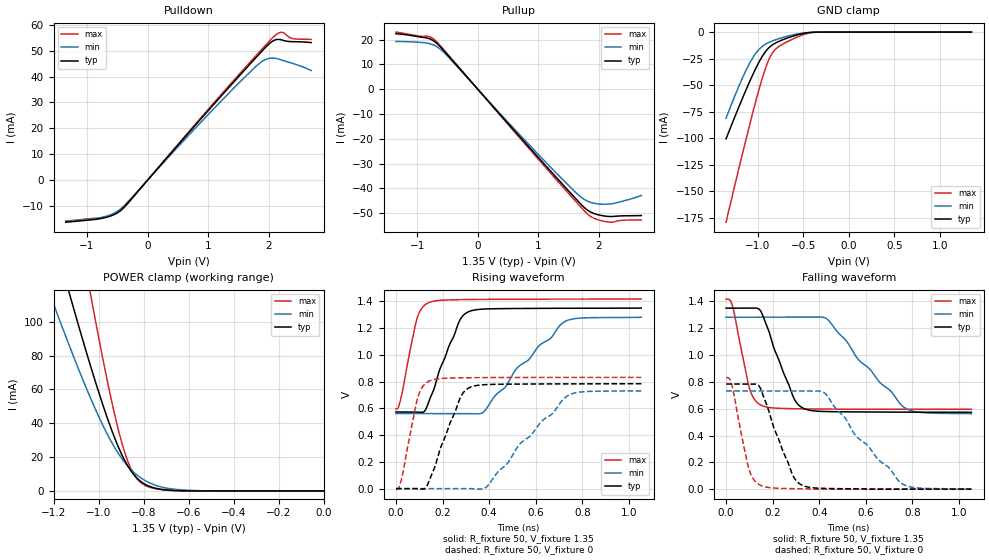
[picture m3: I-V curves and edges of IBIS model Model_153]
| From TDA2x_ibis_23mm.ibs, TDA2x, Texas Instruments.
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| Model based on original model for DDR_SEIOPB_H
|   Sub model SR010_DRV34_1P35
[model]   Model_153
|[Description]  [1.35V-I/O-X-X]
|   , ,
|[Input Load]
|[Output Drive]
|Voltage   1.35V
|Mode   I/O
Model_type   I/O
Polarity   Non-Inverting
Enable   Active-Low
Vinl =  0.585
Vinh =  0.765
Cref =  15.0000pF
Rref =  100.0000M
Vref =  0V
Vmeas =  0.675
C_comp   2p   2p   2p
[Model Spec]
Vinl   0.585   0.55125   0.61875
Vinh   0.765   0.73125   0.79875
[Receiver Thresholds]
Tslew_ac = 5n
Vth= 0.675
Vth_max= 0.709
Vth_min= 0.608
Vinh_ac= 0.175
Vinh_dc= 0.1
Vinl_ac= -0.175
Vinl_dc= -0.1
[Temperature Range]   25   125   -40
[Voltage Range]   1.35   1.2825   1.4175
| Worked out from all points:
|   slope of the pulldown table from 0 to 0.203 V, typ, clamps not added: 36.8 ohm
|   slope of the pullup table from 0 to 0.203 V, typ, clamps not added: 36 ohm
|   GND clamp passes 1 mA (typ) near -0.48 V on its own axis
|   POWER clamp passes 1 mA (typ) near -0.72 V on its own axis
|   rising waveform, R_fixture 50, V_fixture 1.35: 20-80 % time 99.6ps typ, 239ps min, 55.7ps max; typ from 0.573 V to 1.35 V
|   rising waveform, R_fixture 50, V_fixture 0: 20-80 % time 98.8ps typ, 233ps min, 55.9ps max; typ from 0 V to 0.784 V
|   falling waveform, R_fixture 50, V_fixture 1.35: 20-80 % time 99ps typ, 221ps min, 57.3ps max; typ from 1.35 V to 0.573 V
|   falling waveform, R_fixture 50, V_fixture 0: 20-80 % time 99.4ps typ, 226ps min, 56.8ps max; typ from 0.784 V to 0 V
[POWER_clamp]
-1.35V    224.4mA    165.8mA    358.5mA
-1.214V   157mA      115.5mA    250.8mA
-1.132V   117.8mA    86.59mA    187.7mA
-1.118V   111.4mA    81.92mA    177.3mA
-1.036V   74.26mA    55.16mA    116.8mA
-954.5mV  40.7mA     31.91mA    61.06mA
-900mV    22.42mA    19.79mA    30.14mA
-859.1mV  12.48mA    13.09mA    13.96mA
-804.5mV  4.85mA     7.084mA    4.132mA
-736.4mV  1.313mA    2.9mA      1.073mA
-627.3mV  101.6uA    577.3uA    45.9uA
0V        75.63nA    322.4nA    418.5nA
[Pulldown]
-1.35V    -16.25mA   -15.93mA   -15.81mA
-736.4mV  -14.67mA   -14.31mA   -14.33mA
-531.8mV  -13.09mA   -12.54mA   -12.91mA
-409.1mV  -10.94mA   -10.36mA   -11.07mA
1.145V    30.69mA    28.89mA    31.23mA
1.718V    45.54mA    42.37mA    46.27mA
1.923V    50.72mA    46.33mA    51.51mA
2.086V    53.98mA    47.12mA    55.52mA
2.209V    54.19mA    46.41mA    57.19mA
2.25V     53.89mA    46.1mA     56.9mA
2.373V    53.5mA     45.23mA    54.8mA
2.7V      53.13mA    42.33mA    54.36mA
[Pullup]
-1.35V    22.33mA    19.2mA     23.01mA
-981.8mV  21.15mA    18.91mA    21.43mA
-818.2mV  20.5mA     18.48mA    21.31mA
-736.4mV  19.62mA    17.88mA    20.36mA
-613.6mV  16.97mA    16.06mA    17.42mA
1.064V    -29.25mA   -27.93mA   -29.99mA
1.555V    -42.46mA   -40.17mA   -43.52mA
1.759V    -47.7mA    -44.45mA   -49.03mA
1.923V    -50.14mA   -45.98mA   -52.07mA
2.127V    -51.21mA   -46.35mA   -53.42mA
2.291V    -51.16mA   -45.77mA   -53.24mA
2.7V      -50.91mA   -42.85mA   -52.71mA
[GND_clamp]
-1.35V    -100.7mA   -81.27mA   -179.3mA
-1.241V   -77.31mA   -57.61mA   -140mA
-1.132V   -54.83mA   -36.31mA   -101.6mA
-1.05V    -39.08mA   -23.36mA   -74mA
-968.2mV  -25.28mA   -14.71mA   -48.34mA
-913.6mV  -18.13mA   -11.32mA   -33.52mA
-859.1mV  -13.28mA   -9.024mA   -22.35mA
-831.8mV  -11.61mA   -8.091mA   -18.64mA
-777.3mV  -9.078mA   -6.444mA   -14.07mA
-531.8mV  -1.871mA   -1.307mA   -3.441mA
-368.2mV  -88.76uA   -111.2uA   -158uA
1.35V     75.63nA    385.5nA    349.4nA
[Ramp]
dV/dt_f 0.46668874/99.146569p 0.43376197/0.22156618n  0.4935505/57.34186p
dV/dt_r 0.47306492/99.33325p  0.44203139/0.23464204n 0.50172483/56.138411p
R_load = 50
[Rising Waveform]
R_fixture = 50
V_fixture = 1.35
V_fixture_min = 1.2825
V_fixture_max = 1.4175
0s        573.3mV    561.4mV    596.7mV
23.37ps   572.5mV    561.3mV    689.6mV
90.39ps   572.2mV    561.3mV    1.272V
139.6ps   643.8mV    561.3mV    1.39V
269.5ps   1.242V     561.2mV    1.413V
312.7ps   1.324V     560.1mV    1.414V
377.8ps   1.343V     575.3mV    1.415V
518.6ps   1.347V     899.5mV    1.417V
723.4ps   1.349V     1.248V     1.417V
1.053ns   1.35V      1.282V     1.417V
[Rising Waveform]
R_fixture = 50
V_fixture = 0
V_fixture_min = 0
V_fixture_max = 0
485fs     0V         0V         0V
26.19ps   0V         0V         86.87mV
94.99ps   0V         0V         688.4mV
142.6ps   58.39mV    0V         804.3mV
273.9ps   670.9mV    0V         828.4mV
317.3ps   756.9mV    0V         829.4mV
389.8ps   778.1mV    14.4mV     830.5mV
531.4ps   781.9mV    332.7mV    831.5mV
736.9ps   783.4mV    694.8mV    832mV
1.053ns   784.4mV    732.7mV    832.1mV
[Falling Waveform]
R_fixture = 50
V_fixture = 1.35
V_fixture_min = 1.2825
V_fixture_max = 1.4175
0s        1.35V      1.282V     1.417V
28.71ps   1.35V      1.283V     1.36V
103.3ps   1.35V      1.283V     737.6mV
154.2ps   1.31V      1.283V     622.9mV
288.3ps   689mV      1.282V     600.1mV
331.6ps   603.4mV    1.282V     598.9mV
436.1ps   578.7mV    1.265V     597.3mV
568ps     576mV      967mV      596.3mV
772.9ps   574.4mV    600.4mV    595.8mV
1.053ns   573.3mV    561.4mV    595.7mV
[Falling Waveform]
R_fixture = 50
V_fixture = 0
V_fixture_min = 0
V_fixture_max = 0
485fs     784.4mV    732.7mV    832.1mV
26.2ps    784.6mV    732.7mV    769.2mV
99.35ps   784.1mV    732.8mV    142.5mV
146.8ps   754.8mV    732.8mV    29.45mV
284.5ps   111.1mV    732.7mV    3.865mV
326ps     29.8mV     732.5mV    2.709mV
426.1ps   5.385mV    712.9mV    0V
557.4ps   2.509mV    397.1mV    0V
757.3ps   0V         38.71mV    0V
1.053ns   0V         0V         0V
